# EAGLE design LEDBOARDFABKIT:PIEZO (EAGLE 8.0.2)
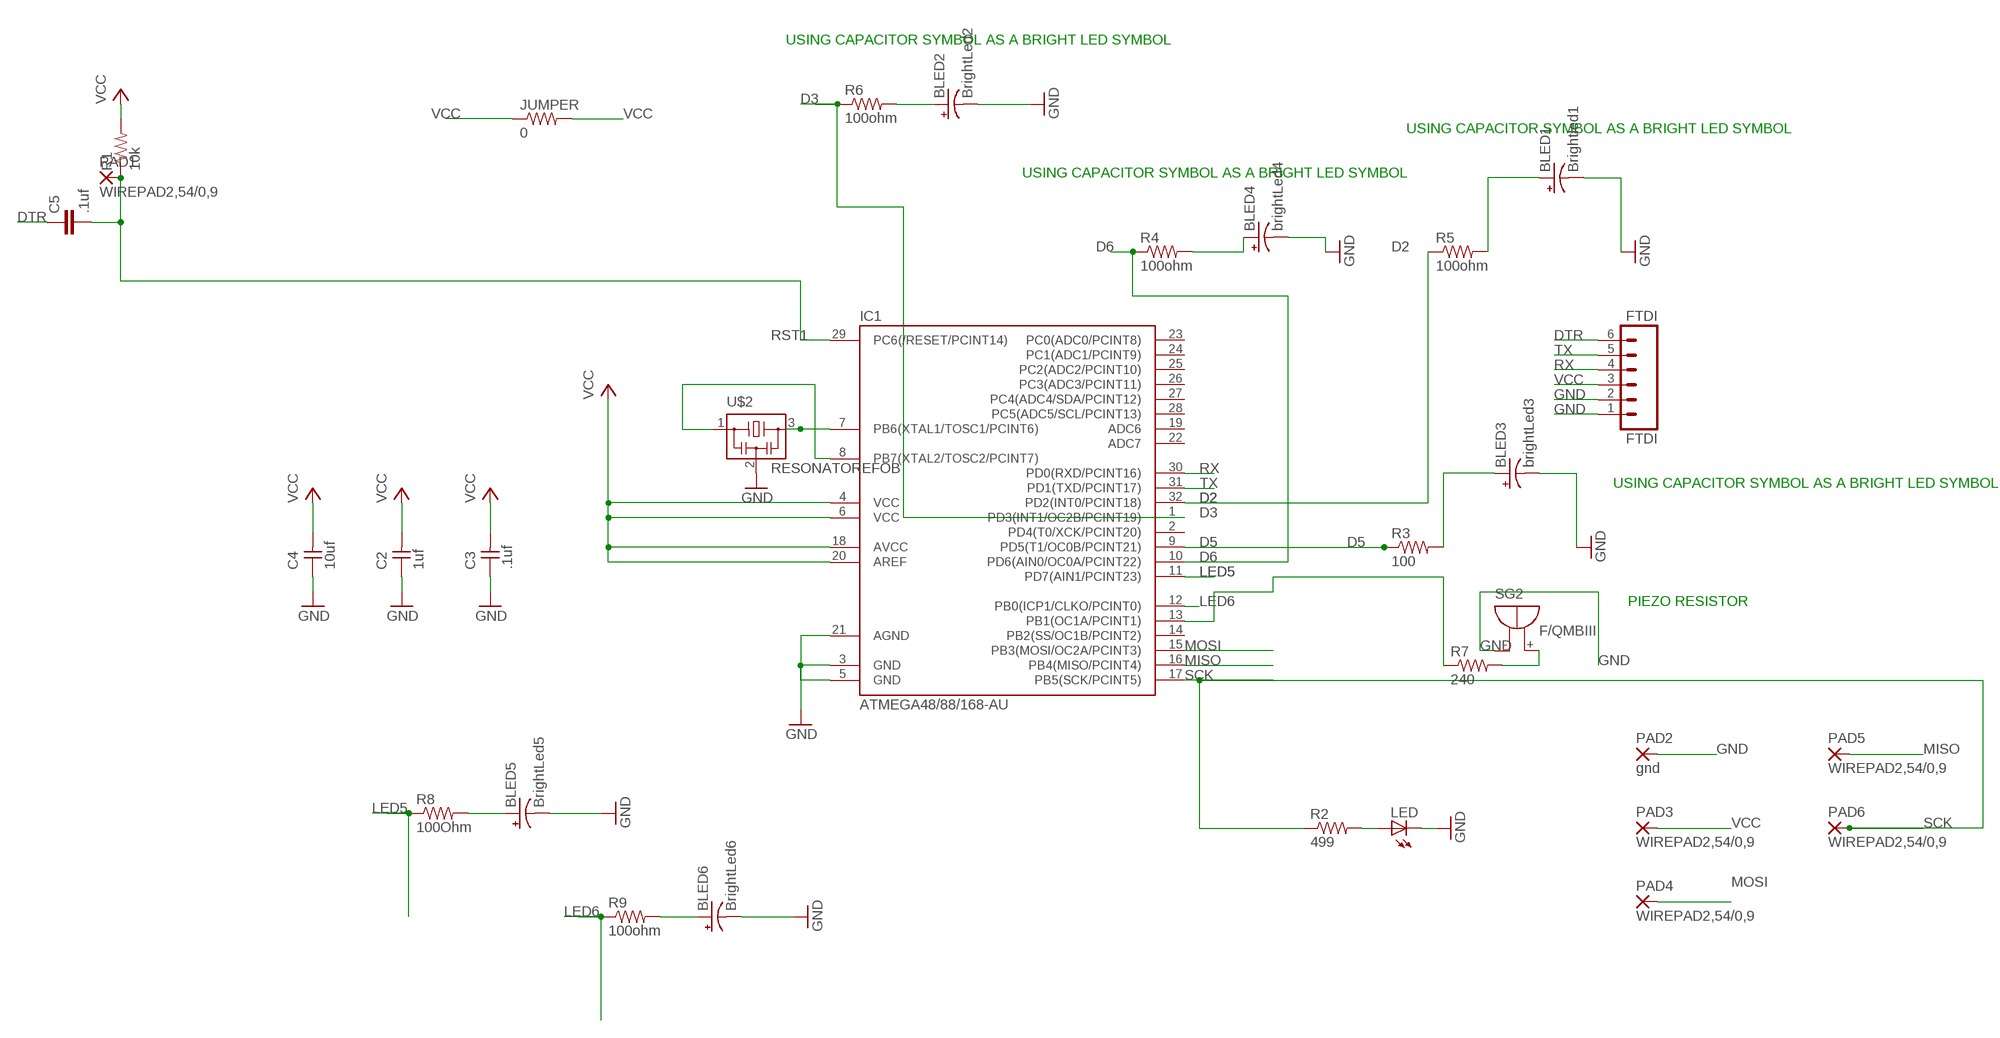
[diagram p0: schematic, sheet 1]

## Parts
BLED1  Brightled1  CAP_POL3528  [EIA3528]
BLED2  BrightLed2  CAP_POL3528  [EIA3528]
BLED3  brightLed3  CAP_POL3528  [EIA3528]
BLED4  brightLed4  CAP_POL3528  [EIA3528]
BLED5  BrightLed5  CAP_POL3528  [EIA3528]
BLED6  BrightLed6  CAP_POL3528  [EIA3528]
C2  1uf  UNPOLARIZED_CAPACITOR1206  [1206]
C3  .1uf  UNPOLARIZED_CAPACITOR1206  [1206]
C4  10uf  UNPOLARIZED_CAPACITOR1206  [1206]
C5  .1uf  C-EUC1206  [C1206]
FTDI  FTDI  M06SMD  [1X06-SMD]
IC1  ATMEGA48/88/168-AU  [TQFP32-08]
JUMPER  0  RES-US1206FAB  [R1206FAB]
LED  LED1206  [1206]
PAD1  WIREPAD2,54/0,9  [2,54/0,9]
PAD2  gnd  WIREPAD2,54/0,9  [2,54/0,9]
PAD3  WIREPAD2,54/0,9  [2,54/0,9]
PAD4  WIREPAD2,54/0,9  [2,54/0,9]
PAD5  WIREPAD2,54/0,9  [2,54/0,9]
PAD6  WIREPAD2,54/0,9  [2,54/0,9]
R1  10k  RESISTOR1206  [1206]
R2  499  RESISTOR1206  [1206]
R3  100  RES-US1206FAB  [R1206FAB]
R4  100ohm  RES-US1206FAB  [R1206FAB]
R5  100ohm  RES-US1206FAB  [R1206FAB]
R6  100ohm  RES-US1206FAB  [R1206FAB]
R7  240  RES-US1206FAB  [R1206FAB]
R8  100Ohm  RES-US1206FAB  [R1206FAB]
R9  100ohm  RES-US1206FAB  [R1206FAB]
SG2  F/QMBIII  [F/QMBIII]
U$2  RESONATOREFOB  [EFOBM]

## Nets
D2: IC1.32(PD2(INT0/PCINT18)) R5.1
D3: IC1.1(PD3(INT1/OC2B/PCINT19)) R6.1
D5: IC1.9(PD5(T1/OC0B/PCINT21)) R3.1
D6: IC1.10(PD6(AIN0/OC0A/PCINT22)) R4.1
DTR: C5.1 FTDI.6
GND: BLED1.C(-) BLED2.C(-) BLED3.C(-) BLED4.C(-) BLED5.C(-) BLED6.C(-) C2.1 C3.1 C4.1 FTDI.1 FTDI.2 IC1.3(GND) IC1.5(GND) IC1.21(AGND) LED.2(C) PAD2.1(P) SG2.-(+) U$2.2
LED5: IC1.11(PD7(AIN1/PCINT23)) R8.1
LED6: IC1.12(PB0(ICP1/CLKO/PCINT0)) R9.1
MISO: IC1.16(PB4(MISO/PCINT4)) PAD5.1(P)
MOSI: IC1.15(PB3(MOSI/OC2A/PCINT3)) PAD4.1(P)
N$1: IC1.8(PB7(XTAL2/TOSC2/PCINT7)) U$2.1
N$3: R7.2 SG2.+(-)
N$4: BLED4.A(+) R4.2
N$5: BLED3.A(+) R3.2
N$6: BLED1.A(+) R5.2
N$7: IC1.13(PB1(OC1A/PCINT1)) R7.1
N$8: BLED2.A(+) R6.2
N$9: IC1.7(PB6(XTAL1/TOSC1/PCINT6)) U$2.3
N$10: BLED5.A(+) R8.2
N$11: BLED6.A(+) R9.2
N$23: LED.1(A) R2.2
RST1: C5.2 IC1.29(PC6(/RESET/PCINT14)) PAD1.1(P) R1.1
RX: FTDI.4 IC1.30(PD0(RXD/PCINT16))
SCK: IC1.17(PB5(SCK/PCINT5)) PAD6.1(P) R2.1
TX: FTDI.5 IC1.31(PD1(TXD/PCINT17))
VCC: C2.2 C3.2 C4.2 FTDI.3 IC1.4(VCC) IC1.6(VCC) IC1.18(AVCC) IC1.20(AREF) JUMPER.1 JUMPER.2 PAD3.1(P) R1.2
Unconnected: IC1.2(PD4(T0/XCK/PCINT20)) IC1.14(PB2(SS/OC1B/PCINT2)) IC1.19(ADC6) IC1.22(ADC7) IC1.23(PC0(ADC0/PCINT8)) IC1.24(PC1(ADC1/PCINT9)) IC1.25(PC2(ADC2/PCINT10)) IC1.26(PC3(ADC3/PCINT11)) IC1.27(PC4(ADC4/SDA/PCINT12)) IC1.28(PC5(ADC5/SCL/PCINT13))

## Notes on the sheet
- USING CAPACITOR SYMBOL AS A BRIGHT LED SYMBOL
- USING CAPACITOR SYMBOL AS A BRIGHT LED SYMBOL
- USING CAPACITOR SYMBOL AS A BRIGHT LED SYMBOL
- USING CAPACITOR SYMBOL AS A BRIGHT LED SYMBOL
- PIEZO RESISTOR

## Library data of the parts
BLED1-BLED6 = 00_SparkFun:CAP_POL: Capacitor Polarized
C2-C4 = ng:UNPOLARIZED_CAPACITOR: unpolarized_capacitor
C5 = rcl:C-EU: CAPACITOR, European symbol
FTDI = SparkFun:M06: Header 6 Standard 6-pin 0.1" header. Use with straight break away headers (SKU : PRT-00116), right angle break away headers (PRT-00553), swiss pins (PRT-00743), machine pins (PRT-00117), and female headers (PRT-00115). Molex polarized connector foot print use with SKU : PRT-08094 with associated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
IC1 = atmega8:ATMEGA48/88/168
JUMPER R3-R9 = fab:RES-US: Resistor (US Symbol)
LED = ng:LED
PAD1-PAD6 = wirepad:WIREPAD: Wire PAD connect wire on PCB
R1 R2 = ng:RESISTOR
SG2 = buzzer:F/QMBIII: BUZZER; OC_FARNELL: unknown; OC_NEWARK: unknown
U$2 = fab:RESONATOR

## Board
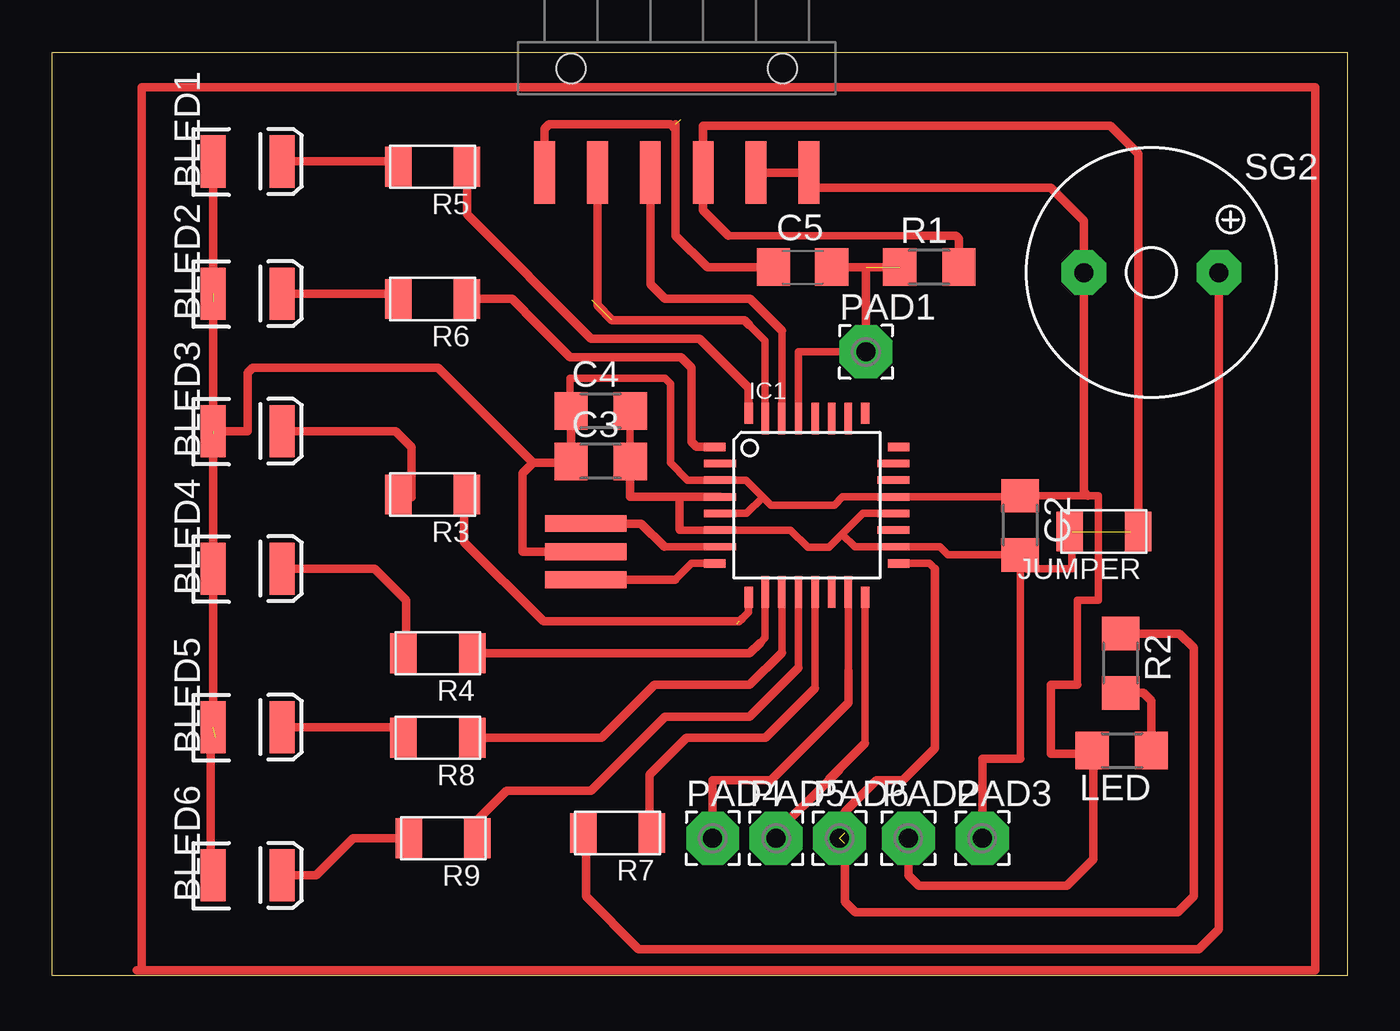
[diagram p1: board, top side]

Size 62.26 x 44.37 mm. Coordinates in mm from the lower left corner, seen from the top.
Outline: 0,44.37 62.25,44.37 62.25,0 0,0 0,44.37
Copper layers (1*16): Top 0.035mm / dielectric 1.5mm / Bottom 0.035mm
Design rules "default *": minimum track width 10mil, minimum drill 24mil, track to track 16mil, track to pad 16mil, pad to pad 16mil, via to via 16mil, smd to smd 16mil, copper to edge 16mil, drill to drill 8mil, minimum pad ring 10mil, minimum via ring 8mil, stop-mask expansion 4mil, vias tented up to drill 0mil, thermal gap 10mil

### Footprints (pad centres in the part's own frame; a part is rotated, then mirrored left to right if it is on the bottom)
EIA3528 = smd 1.2 x 2.5: A 1.65,0; C -1.65,0
1206 = smd 1.6 x 1.803: 1 -1.422,0; 2 1.422,0
C1206 = smd 1.6 x 1.8: 1 -1.4,0; 2 1.4,0
1X06-SMD = smd 1 x 3: 1 -6.35,5; 2 -3.81,5; 3 -1.27,5; 4 1.27,5; 5 3.81,5; 6 6.35,5 | hole 1.4: -5.08,0; 5.08,0
TQFP32-08 = smd 1.016 x 0.406: 1 -4.42,2.8; 8 -4.42,-2.8; 17 4.42,-2.8; 24 4.42,2.8 | smd 1.524 x 0.356: 2 -4.166,2; 3 -4.166,1.2; 4 -4.166,0.4; 5 -4.166,-0.4; 6 -4.166,-1.2; 7 -4.166,-2; 18 4.166,-2; 19 4.166,-1.2; 20 4.166,-0.4; 21 4.166,0.4; 22 4.166,1.2; 23 4.166,2 | smd 0.406 x 1.016: 9 -2.8,-4.42; 16 2.8,-4.42; 25 2.8,4.42; 32 -2.8,4.42 | smd 0.356 x 1.524: 10 -2,-4.166; 11 -1.2,-4.166; 12 -0.4,-4.166; 13 0.4,-4.166; 14 1.2,-4.166; 15 2,-4.166; 26 2,4.166; 27 1.2,4.166; 28 0.4,4.166; 29 -0.4,4.166; 30 -1.2,4.166; 31 -2,4.166
R1206FAB = smd 1.27 x 1.905: 1 -1.651,0; 2 1.651,0
2,54/0,9 = drill 0.914 pad 2.54 octagon: 1 0,0
F/QMBIII = drill 0.914 pad 2.159 octagon: + 3.251,0; - -3.251,0
EFOBM = smd 0.8 x 3.9: 1 -1.35,0; 2 0,0; 3 1.35,0

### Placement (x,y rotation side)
BLED1  9.4,39.12 0 top
BLED2  9.4,32.77 0 top
BLED3  9.4,26.16 0 top
BLED4  9.4,19.56 0 top
BLED5  9.4,11.94 0 top
BLED6  9.4,4.83 0 top
C2  46.53,21.64 270 top
C3  26.37,24.71 0 top
C4  26.37,27.13 0 top
C5  36.07,34.04 0 top
FTDI  30.02,43.59 180 top
IC1  36.27,22.61 0 top
JUMPER  50.55,21.34 180 top
LED  51.41,10.82 180 top
PAD1  39.12,29.97 0 top
PAD2  41.15,6.6 0 top
PAD3  44.7,6.6 0 top
PAD4  31.75,6.6 0 top
PAD5  34.8,6.6 0 top
PAD6  37.85,6.6 0 top
R1  42.16,34.04 0 top
R2  51.36,15.01 270 top
R3  18.29,23.11 180 top
R4  18.54,15.49 180 top
R5  18.29,38.86 180 top
R6  18.29,32.51 180 top
R7  27.18,6.86 180 top
R8  18.54,11.43 180 top
R9  18.8,6.6 180 top
SG2  52.83,33.78 0 top
U$2  25.65,20.37 90 top

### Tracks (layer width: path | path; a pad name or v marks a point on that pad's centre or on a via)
D2
  Top 0.406: 19.81,38.73 R5.1 | IC1.32 33.47,28.25 31.12,30.61 25.91,30.61 19.94,36.58 | 19.94,36.58 R5.1 | R5.1 19.94,36.58
D3
  Top 0.406: 23.37,31.24 22.1,32.51 | 23.37,31.24 24.89,29.72 30.23,29.72 30.73,29.21 30.73,25.65 30.98,25.41 IC1.1 | R6.1 22.1,32.51 | 22.1,32.51 23.37,31.24
D5  (1 unrouted)
  Top 0.356: IC1.9 33.47,17.47 33.15,17.14
  Top 0.406: 33.15,17.14 33.02,17.02 23.62,17.02 19.81,20.83 19.81,22.99 R3.1
D6
  Top 0.356: 34.04,16 34.27,16.24 IC1.10
  Top 0.406: R4.1 33.53,15.49 34.04,16
DTR  (1 unrouted)
  Top 0.356: 23.37,37.88 FTDI.6 23.37,37.82 23.37,37.88
  Top 0.406: C5.1 31.5,34.04 29.97,35.56 29.97,40.64 | 29.97,40.64 29.97,40.89 | FTDI.6 23.67,40.69 23.88,40.89 29.72,40.89 29.97,40.64
GND  (3 unrouted)
  Top 0.356: C4.1 24.89,27.18 24.89,28.7 29.46,28.7 29.72,28.45 29.72,24.64 30.55,23.81 IC1.3 33.34,23.81 34.16,22.99 | 34.16,22.99 34.54,22.61 37.59,22.61 37.99,23.01 IC1.21 46.48,23.01 C2.1 49.78,23.06 50.29,23.06 50.29,18.03 49.28,18.03 49.28,13.97 | IC1.5 33.38,22.21 34.16,22.99
  Top 0.406: 24.97,27.41 C4.1 C3.1 24.87,24.64 23.11,24.64 | 47.04,22.86 C2.1 46.48,23.11 | PAD2.1 41.15,4.83 41.66,4.32 48.77,4.32 50.04,5.59 50.04,10.77 | 49.28,13.97 48.01,13.97 48.01,10.67 49.94,10.67 | 49.94,10.67 49.99,10.67 LED.2 50.04,10.77 | FTDI.2 FTDI.1 36.14,37.85 48.01,37.85 49.58,36.27 SG2.- 49.58,23.27 49.78,23.06 | 49.94,10.67 50.04,10.77 | 23.11,24.64 22.61,24.13 22.61,20.37 U$2.2 | 7.75,32.39 7.62,32.26 | 7.87,25.65 7.62,25.91 7.75,26.04 BLED2.C BLED1.C | 7.87,11.43 7.62,11.18 7.62,4.95 BLED6.C | BLED5.C BLED4.C BLED3.C 9.4,26.16 9.4,28.96 9.65,29.21 11.94,29.21 12.45,29.21 18.54,29.21 23.11,24.64
LED5
  Top 0.356: IC1.11 35.07,15.51
  Top 0.406: 35.07,15.51 33.53,13.97 28.96,13.97 26.42,11.43 R8.1
LED6
  Top 0.356: IC1.12 35.87,14.79
  Top 0.406: R9.1 20.45,7.49 21.84,8.89 25.91,8.89 29.46,12.45 33.53,12.45 35.87,14.79
MISO
  Top 0.356: 39.07,11.18 IC1.16
  Top 0.406: PAD5.1 34.8,6.86 37.34,9.4 | 37.85,9.91 37.34,9.4 | 37.34,9.4 37.34,9.44 39.07,11.18
MOSI
  Top 0.356: IC1.15 38.27,14.65
  Top 0.406: PAD4.1 31.75,9.4 34.54,9.4 38.27,13.12 38.27,14.65
N$1
  Top 0.356: IC1.8 30.73,19.81 29.97,19.05 | 27.21,19.05 U$2.1
  Top 0.406: U$2.1 29.94,19.02 29.97,19.05
N$3
  Top 0.406: SG2.+ 56.08,3.3 | 56.08,3.3 56.08,2.24 | R7.2 25.65,6.73 25.65,3.81 28.19,1.27 55.12,1.27 56.08,2.24 | 56.08,3.3 56.08,2.24
N$4
  Top 0.406: BLED4.A 15.49,19.56 17.02,18.03 17.02,15.62 R4.2
N$5
  Top 0.406: BLED3.A 16.51,26.16 17.27,25.4 17.27,22.99 R3.2
N$6
  Top 0.406: BLED1.A 16.38,39.12 R5.2
N$7
  Top 0.356: IC1.13 36.67,13.81
  Top 0.406: 36.67,13.81 34.29,11.43 30.48,11.43 28.7,9.65 28.7,6.98 R7.1
N$8
  Top 0.406: BLED2.A 16.38,32.77 R6.2
N$9
  Top 0.356: 29.43,20.61 IC1.7 | 25.79,21.59 U$2.3
  Top 0.406: U$2.3 28.32,21.72 29.43,20.61
N$10
  Top 0.406: 16.38,11.94 R8.2 16.38,11.94 | BLED5.A 16.38,11.94
N$11
  Top 0.406: BLED6.A 12.7,4.83 14.48,6.6 17.02,6.6 17.53,6.1 17.53,6.22 R9.2
N$12
  Top 0.406: 4.06,0.25 4.32,0.25 | 4.32,0.25 60.71,0.25 60.71,42.67 4.32,42.67 4.32,0.25
N$23
  Top 0.356: LED.1 53.09,11.07
  Top 0.406: R2.2 52.45,13.59 52.83,13.21 LED.1
RST1  (1 unrouted)
  Top 0.356: PAD1.1 35.87,29.97 IC1.29
  Top 0.406: 39.12,34.04 PAD1.1 | C5.2 R1.1
RX
  Top 0.356: 35.07,30.99 IC1.30
  Top 0.406: 28.45,37.77 FTDI.4 28.75,33.22 29.46,32.51 33.55,32.51 35.07,30.99
SCK  (2 unrouted)
  Top 0.356: IC1.17 42.17,19.81 42.42,19.56
  Top 0.406: 42.42,19.56 42.42,10.92 40.89,9.4 39.62,9.4 38.1,7.87 38.1,6.86 | R2.1 54.18,16.43 54.86,15.75 54.86,3.81 54.1,3.05 38.61,3.05 38.1,3.56 38.1,6.35
TX  (1 unrouted)
  Top 0.356: 25.91,37.77 FTDI.5 | IC1.31 34.27,30.5 33.53,31.24
  Top 0.406: 33.53,31.24 33.27,31.5 26.92,31.5 26.21,32.21 FTDI.5
VCC  (1 unrouted)
  Top 0.356: 30.18,21.41 30.15,21.44 30.15,21.41 IC1.6 35.49,21.41 36.32,20.57 37.34,20.57 37.97,21.21 | 41.81,35.56 32.51,35.56 | C4.2 C3.2 | JUMPER.2 49.02,21.34 49.02,19.56 46.84,19.56 | 52.32,21.34 JUMPER.1 51.82,21.34 | 46.43,20.32 C2.2 | IC1.20 38.97,22.21 37.97,21.21 | 37.97,21.21 38.58,20.61 IC1.18 42.67,20.61 43.06,20.22 C2.2 | 46.53,10.41 C2.2
  Top 0.406: IC1.4 30.15,23.01 | 30.15,21.44 30.15,23.01 | 30.15,23.01 27.79,23.01 C3.2 | C2.2 46.84,20.22 46.84,19.56 | PAD3.1 44.7,10.41 46.53,10.41 | FTDI.3 31.04,38.61 31.24,38.81 | JUMPER.1 52.2,39.5 50.85,40.84 31.29,40.84 FTDI.3 | FTDI.3 31.29,36.78 32.51,35.56 | R1.2 43.59,35.41 43.43,35.56 41.81,35.56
